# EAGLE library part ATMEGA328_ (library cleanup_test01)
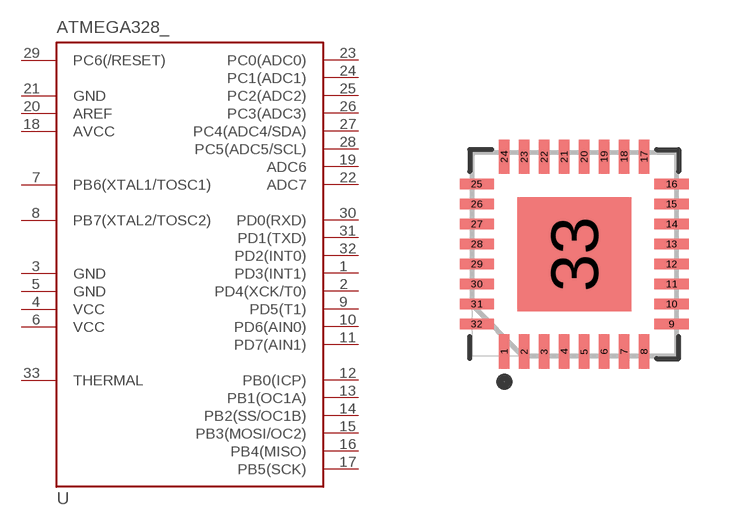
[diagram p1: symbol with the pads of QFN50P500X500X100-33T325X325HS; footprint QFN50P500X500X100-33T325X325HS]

Designator prefix -

## ATMEGA328_32MLF  [QFN50P500X500X100-33T325X325HS]
1  PD3(INT1)
2  PD4(XCK/T0)
3  GND  pwr
4  VCC  pwr
5  GND  pwr
6  VCC  pwr
7  PB6(XTAL1/TOSC1)
8  PB7(XTAL2/TOSC2)
9  PD5(T1)
10  PD6(AIN0)
11  PD7(AIN1)
12  PB0(ICP)
13  PB1(OC1A)
14  PB2(SS/OC1B)
15  PB3(MOSI/OC2)
16  PB4(MISO)
17  PB5(SCK)
18  AVCC  pwr
19  ADC6
20  AREF  pas
21  GND  pwr
22  ADC7
23  PC0(ADC0)
24  PC1(ADC1)
25  PC2(ADC2)
26  PC3(ADC3)
27  PC4(ADC4/SDA)
28  PC5(ADC5/SCL)
29  PC6(/RESET)
30  PD0(RXD)
31  PD1(TXD)
32  PD2(INT0)
33  THERMAL  pas

## Footprint QFN50P500X500X100-33T325X325HS (pad centres in mm)
smd 0.26 x 0.86: 1 -1.75,-2.435; 2 -1.25,-2.435; 3 -0.75,-2.435; 4 -0.25,-2.435; 5 0.25,-2.435; 6 0.75,-2.435; 7 1.25,-2.435; 8 1.75,-2.435; 17 1.75,2.435; 18 1.25,2.435; 19 0.75,2.435; 20 0.25,2.435; 21 -0.25,2.435; 22 -0.75,2.435; 23 -1.25,2.435; 24 -1.75,2.435
smd 0.86 x 0.26: 9 2.435,-1.75; 10 2.435,-1.25; 11 2.435,-0.75; 12 2.435,-0.25; 13 2.435,0.25; 14 2.435,0.75; 15 2.435,1.25; 16 2.435,1.75; 25 -2.435,1.75; 26 -2.435,1.25; 27 -2.435,0.75; 28 -2.435,0.25; 29 -2.435,-0.25; 30 -2.435,-0.75; 31 -2.435,-1.25; 32 -2.435,-1.75
smd 2.85 x 2.85: 33 0,0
